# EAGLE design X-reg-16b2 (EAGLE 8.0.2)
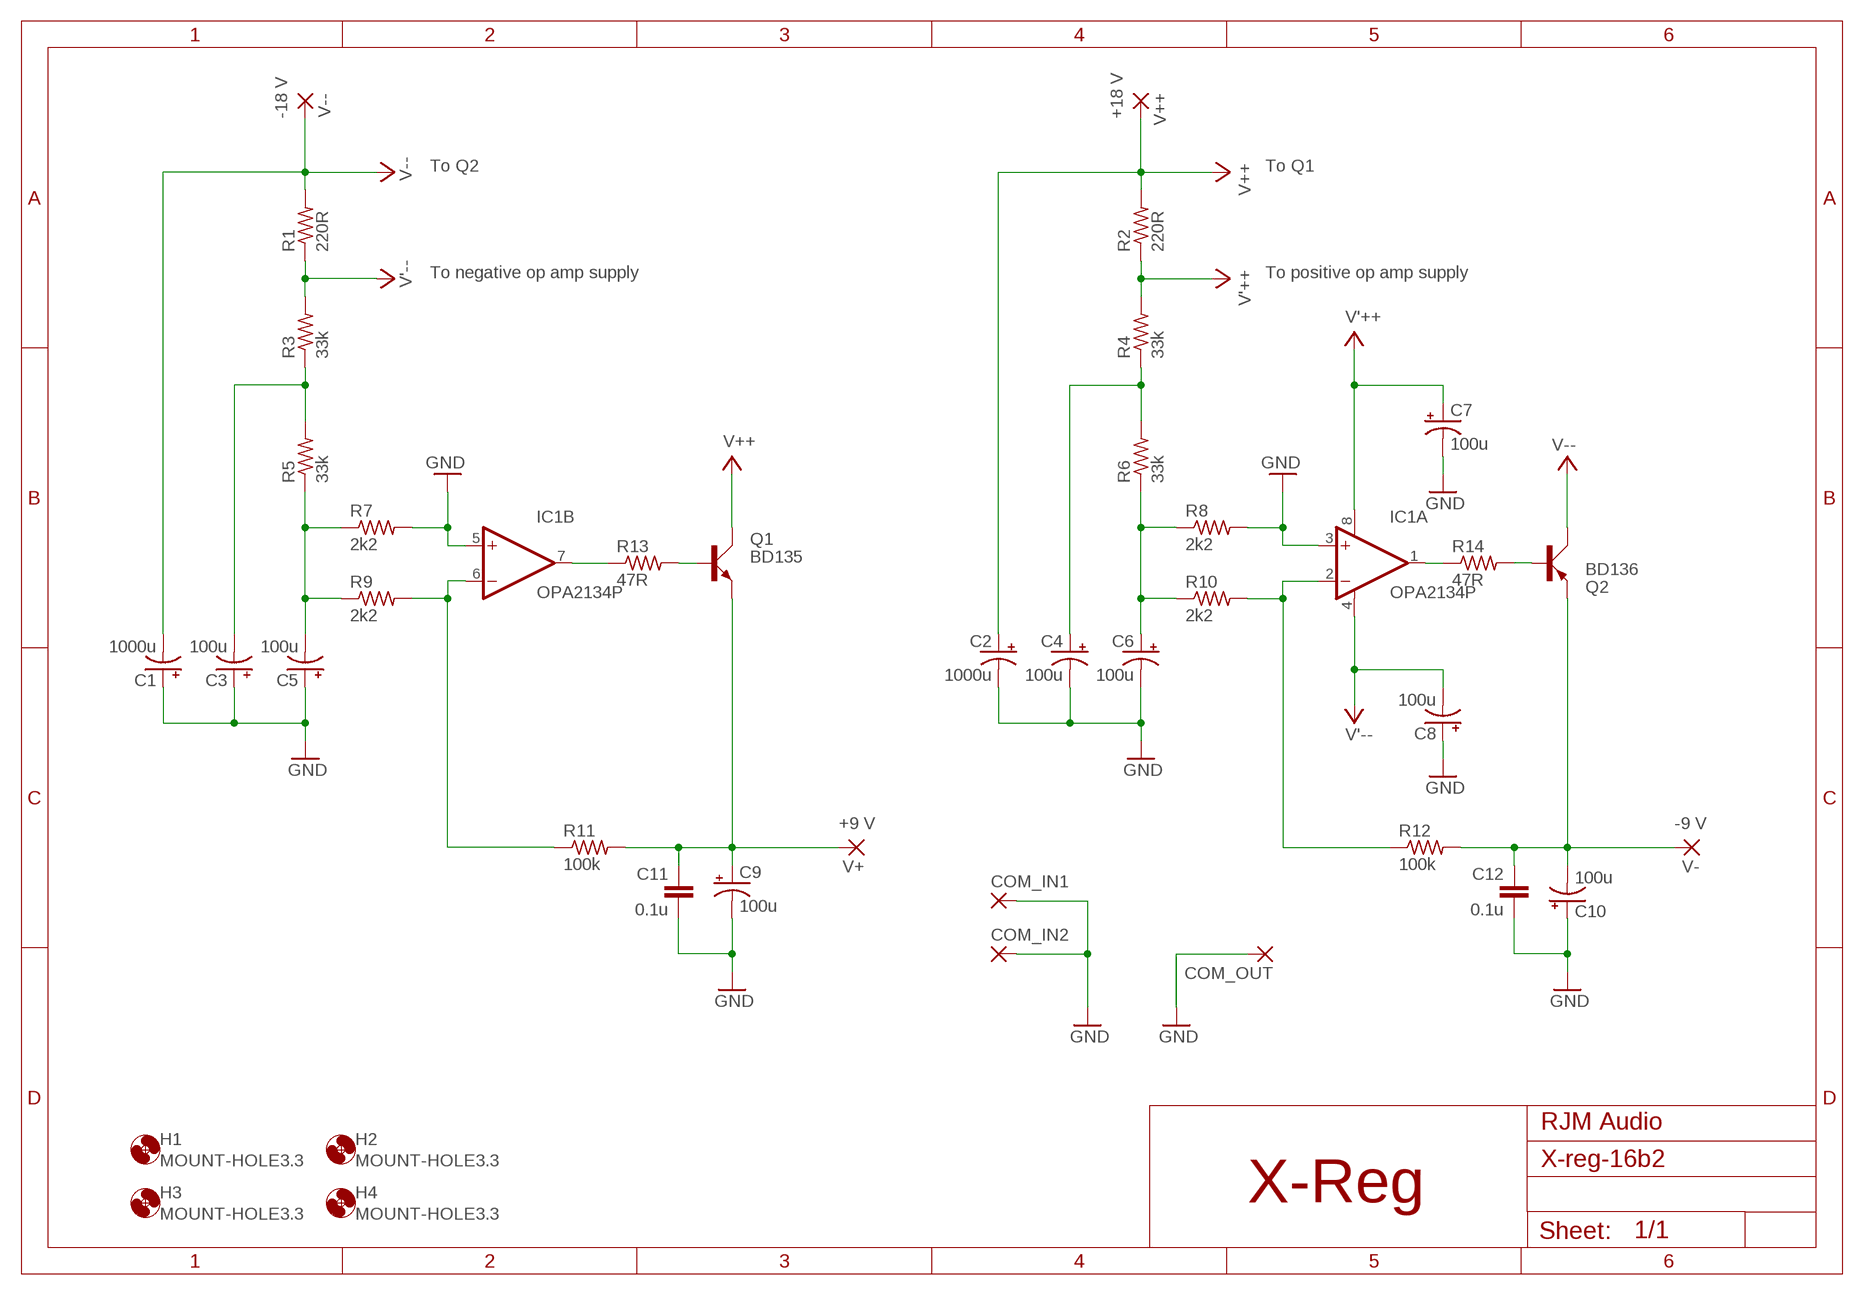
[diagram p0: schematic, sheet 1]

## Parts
C1  1000u  CPOL-USE5-10.5  [E5-10,5]
C2  1000u  CPOL-USE5-10.5  [E5-10,5]
C3  100u  CPOL-USE2.5-6  [E2,5-6]
C4  100u  CPOL-USE2.5-6  [E2,5-6]
C5  100u  CPOL-USE2.5-6  [E2,5-6]
C6  100u  CPOL-USE2.5-6  [E2,5-6]
C7  100u  CPOL-USE2.5-6  [E2,5-6]
C8  100u  CPOL-USE2.5-6  [E2,5-6]
C9  100u  CPOL-USE2.5-6  [E2,5-6]
C10  100u  CPOL-USE2.5-6  [E2,5-6]
C11  0.1u  C-EU050-024X044  [C050-024X044]
C12  0.1u  C-EU050-024X044  [C050-024X044]
COM_IN1  3,17/1,3  [3,17/1,3]
COM_IN2  3,17/1,3  [3,17/1,3]
COM_OUT  3,17/1,3  [3,17/1,3]
H1  MOUNT-HOLE3.3  [3,3]
H2  MOUNT-HOLE3.3  [3,3]
H3  MOUNT-HOLE3.3  [3,3]
H4  MOUNT-HOLE3.3  [3,3]
IC1  OPA2134P  [DIL08]
Q1  BD135  BD139  [TO126AV]
Q2  BD136  BD140  [TO126AV]
R1  220R  R-US_0207/10  [0207/10]
R2  220R  R-US_0207/10  [0207/10]
R3  33k  R-US_0207/10  [0207/10]
R4  33k  R-US_0207/10  [0207/10]
R5  33k  R-US_0207/10  [0207/10]
R6  33k  R-US_0207/10  [0207/10]
R7  2k2  R-US_0207/10  [0207/10]
R8  2k2  R-US_0207/10  [0207/10]
R9  2k2  R-US_0207/10  [0207/10]
R10  2k2  R-US_0207/10  [0207/10]
R11  100k  R-US_0207/10  [0207/10]
R12  100k  R-US_0207/10  [0207/10]
R13  47R  R-US_0207/10  [0207/10]
R14  47R  R-US_0207/10  [0207/10]
V+  3,17/1,3  [3,17/1,3]
V++  3,17/1,3  [3,17/1,3]
V-  3,17/1,3  [3,17/1,3]
V--  3,17/1,3  [3,17/1,3]

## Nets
GND: C1.+ C2.- C3.+ C4.- C5.+ C6.- C7.- C8.+ C9.- C10.+ C11.2 C12.2 COM_IN1.1(P) COM_IN2.1(P) COM_OUT.1(P) IC1.3(A:+IN) IC1.5(B:+IN) R7.2 R8.2
N$2: IC1.7(B:OUT) R13.1
N$3: Q1.B R13.2
N$4: IC1.1(A:OUT) R14.1
N$5: Q2.B R14.2
V'++: C7.+ IC1.8(A:V+) R2.1 R4.2
V'--: C8.- IC1.4(A:V-) R1.1 R3.2
V+: C9.+ C11.1 Q1.E R11.2 V+.1(P)
V++: C2.+ Q1.C R2.2 V++.1(P)
V+FILTER: C4.+ R4.1 R6.2
V+INV: IC1.2(A:-IN) R10.2 R12.1
V+REF: C6.+ R6.1 R8.1 R10.1
V-: C10.- C12.1 Q2.E R12.2 V-.1(P)
V--: C1.- Q2.C R1.2 V--.1(P)
V-FILTER: C3.- R3.1 R5.2
V-INV: IC1.6(B:-IN) R9.2 R11.1
V-REF: C5.- R5.1 R7.1 R9.1

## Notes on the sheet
- -18 V | +18 V
- To Q2 | To Q1
- To negative op amp supply | To positive op amp supply
- +9 V | -9 V
- RJM Audio
- X-Reg

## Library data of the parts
C1 C2 = resistor:CPOL-US: POLARIZED CAPACITOR, American symbol
C3-C10 = rcl:CPOL-US: POLARIZED CAPACITOR, American symbol
C11 C12 = rcl:C-EU: CAPACITOR, European symbol
COM_IN1 COM_IN2 COM_OUT V+ V++ V- V-- = wirepad:3,17/1,3: THROUGH-HOLE PAD
H1-H4 = holes:MOUNT-HOLE: MOUNTING HOLE with drill center marker
IC1 = burr-brown:OPA2134: Operational Amplifier; MF: TEXAS INSTRUMENTS; MPN: OPA2134PA; OC_FARNELL: 1097574; OC_NEWARK: 74K3897
Q1 = transistor-power:BD139: NPN TRANSISTOR
Q2 = transistor-power:BD140: PNP TRANSISTOR
R1-R14 = rcl:R-US_: RESISTOR, American symbol

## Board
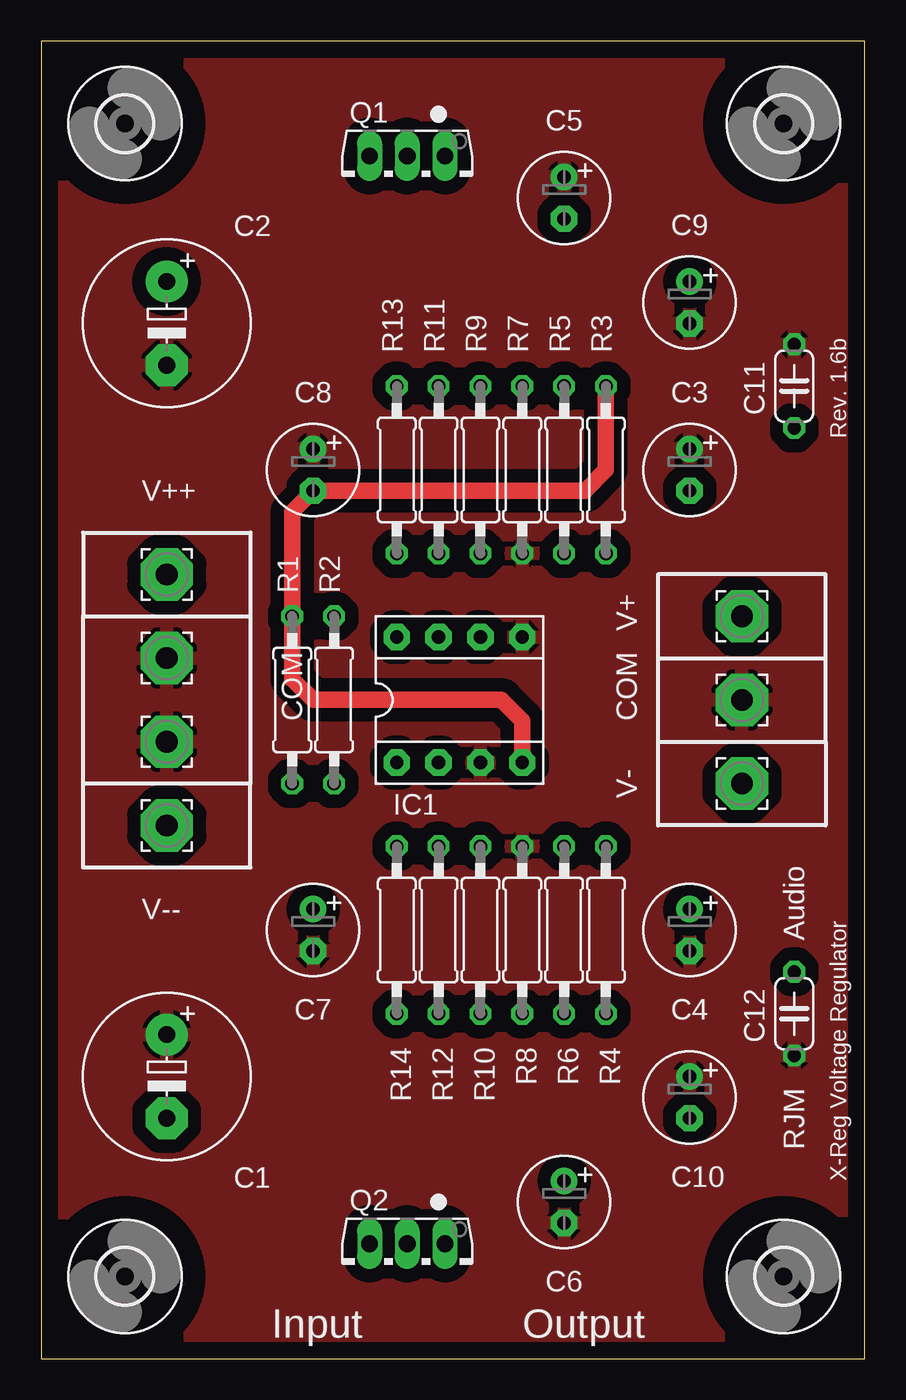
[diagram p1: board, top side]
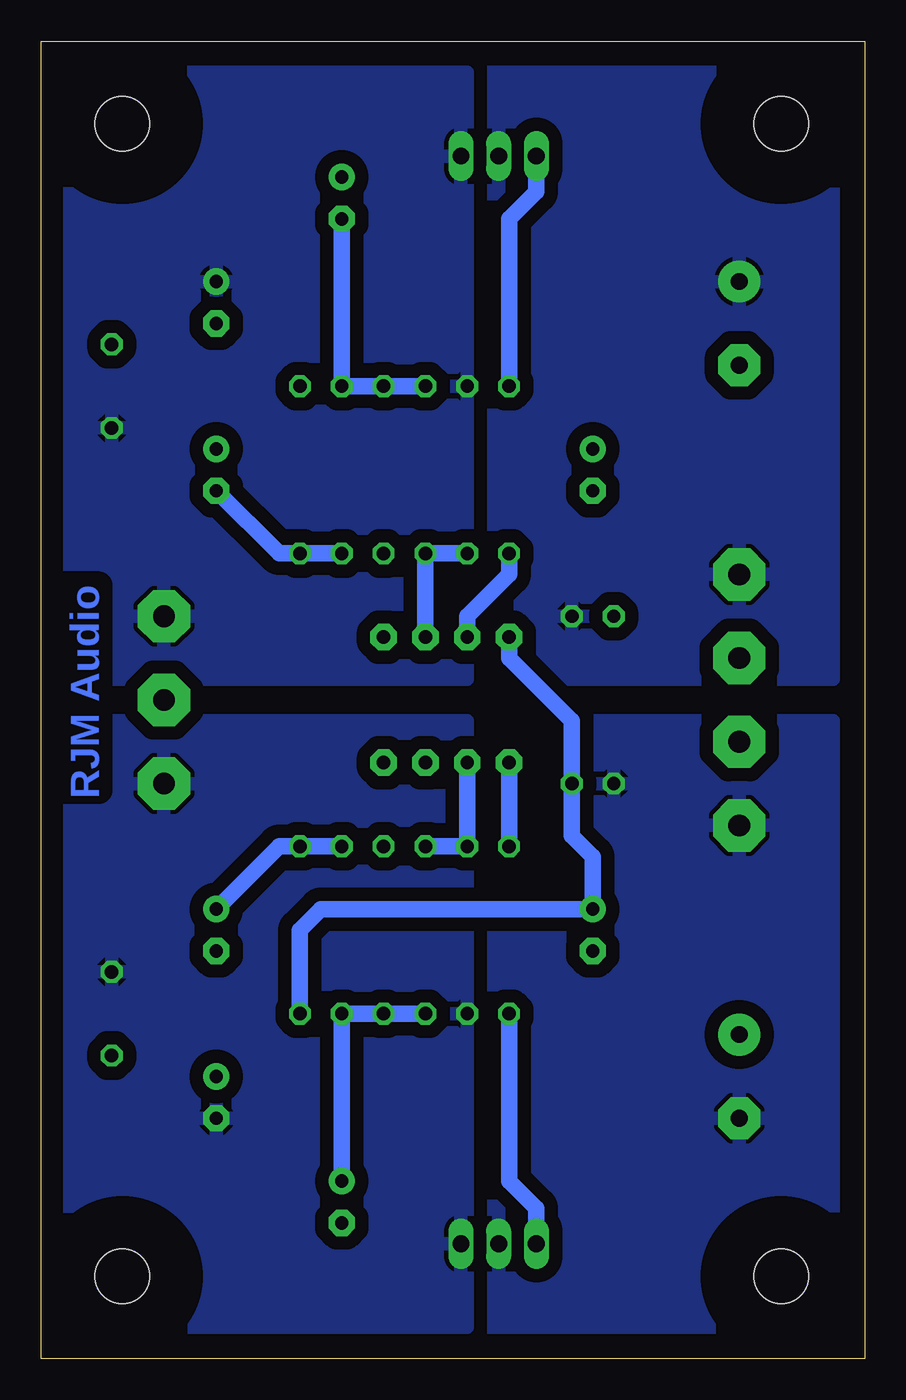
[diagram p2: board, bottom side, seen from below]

Size 50 x 80 mm. Coordinates in mm from the lower left corner, seen from the top.
Outline: 0,0 50,0 50,80 0,80 0,0
Copper layers (1*16): Top 0.035mm / dielectric 1.5mm / Bottom 0.035mm
Design rules "default": minimum track width 10mil, minimum drill 24mil, track to track 8mil, track to pad 8mil, pad to pad 8mil, via to via 8mil, smd to smd 8mil, copper to edge 40mil, drill to drill 8mil, minimum pad ring 10mil, minimum via ring 8mil, stop-mask expansion 4mil, vias tented up to drill 0mil, thermal gap 10mil

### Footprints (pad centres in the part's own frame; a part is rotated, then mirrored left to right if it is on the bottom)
E5-10,5 = drill 1.016 pad 2.54: + -2.54,0 | drill 1.016 pad 2.54 octagon: - 2.54,0
E2,5-6 = drill 0.813 pad 1.6: + -1.27,0 | drill 0.813 pad 1.6 octagon: - 1.27,0
C050-024X044 = drill 0.813 octagon: 1 -2.54,0; 2 2.54,0
3,17/1,3 = drill 1.321 pad 3.175 octagon: 1 0,0
3,3 = hole 3.3: 0,0
DIL08 = drill 0.813 pad 1.6 octagon: 1 -3.81,-3.81; 2 -1.27,-3.81; 3 1.27,-3.81; 4 3.81,-3.81; 5 3.81,3.81; 6 1.27,3.81; 7 -1.27,3.81; 8 -3.81,3.81
TO126AV = drill 1.016 long: B 2.286,-1.27; C 0,-1.27; E -2.286,-1.27
0207/10 = drill 0.813 octagon: 1 -5.08,0; 2 5.08,0

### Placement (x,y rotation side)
C1  7.62,17.14 270 top
C2  7.62,62.87 270 top
C3  39.37,53.98 270 top
C4  39.37,26.04 270 top
C5  31.75,70.48 270 top
C6  31.75,9.53 270 top
C7  16.51,26.04 270 top
C8  16.51,53.98 270 top
C9  39.37,64.13 270 top
C10  39.37,15.88 270 top
C11  45.72,59.05 90 top
C12  45.72,20.95 270 top
COM_IN1  7.62,37.47 0 top
COM_IN2  7.62,42.55 0 top
COM_OUT  42.55,40.01 0 top
H1  5.08,75 0 top
H2  45.08,75 0 top
H3  5.08,5 0 top
H4  45.08,5 0 top
IC1  25.4,40.01 0 top
Q1  22.23,71.75 180 top
Q2  22.23,5.71 180 top
R1  15.24,40.01 270 top
R2  17.78,40.01 90 top
R3  34.29,53.98 90 top
R4  34.29,26.04 270 top
R5  31.75,53.98 270 top
R6  31.75,26.04 90 top
R7  29.21,53.98 270 top
R8  29.21,26.04 90 top
R9  26.67,53.98 270 top
R10  26.67,26.04 90 top
R11  24.13,53.98 90 top
R12  24.13,26.04 270 top
R13  21.59,53.98 90 top
R14  21.59,26.04 270 top
V+  42.55,45.09 0 top
V++  7.62,47.62 0 top
V-  42.55,34.93 0 top
V--  7.62,32.39 0 top

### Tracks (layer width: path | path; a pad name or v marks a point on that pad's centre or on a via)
GND
  pour Top (isolate 0.813): 0,80.01 50.16,80.01 50.16,0 0,0
N$2
  Bottom 1.016: IC1.7 24.13,45.09 21.59,47.62 R13.1
N$3
  Bottom 1.016: R13.2 21.59,69.21 19.94,70.87 Q1.B
N$4
  Bottom 1.016: IC1.1 R14.1
N$5
  Bottom 1.016: Q2.B 19.94,9.14 21.59,10.79 R14.2
V'++
  Bottom 1.016: IC1.8 21.59,42.55 17.78,38.73 R2.1 17.78,31.75 16.51,30.48 C7.+ 33.02,27.3 34.29,26.04 R4.2
V'--
  Top 1.016: R3.2 34.29,53.98 33.02,52.71 C8.- 15.24,51.44 R1.1 15.24,41.27 16.51,40.01 27.94,40.01 29.21,38.73 IC1.4
V+
  pour Bottom (isolate 0.813): 24.13,78.1 24.13,41.27 48.26,41.27 48.26,78.1
V++
  pour Bottom (isolate 0.813, rank 2): 48.26,78.1 1.91,78.1 1.91,41.27 48.26,41.27
  pour Bottom (isolate 0.813, rank 2): 48.26,78.1 1.91,78.1 1.91,41.27 48.26,41.27
V+FILTER
  Bottom 1.016: R6.2 R4.1 35.56,31.11 C4.+
V+INV
  Bottom 1.016: R10.2 R12.1 IC1.2
V+REF
  Bottom 1.016: C6.+ R6.1 R8.1 R10.1
V-
  pour Bottom (isolate 0.813): 24.13,38.73 24.13,1.91 48.26,1.91 48.26,38.73
V--
  pour Bottom (isolate 0.813, rank 2): 48.26,1.91 48.26,38.73 1.91,38.73 1.91,1.91
V-FILTER
  Bottom 1.016: R5.2 R3.1 35.56,48.9 C3.-
V-INV
  Bottom 1.016: R11.1 R9.2 IC1.6
V-REF
  Bottom 1.016: R9.1 R7.1 R5.1 C5.-

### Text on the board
Bottom: RJM Audio
tPlace: Rev. 1.6b | COM | COM | Audio | RJM | X-Reg Voltage Regulator | Input | Output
